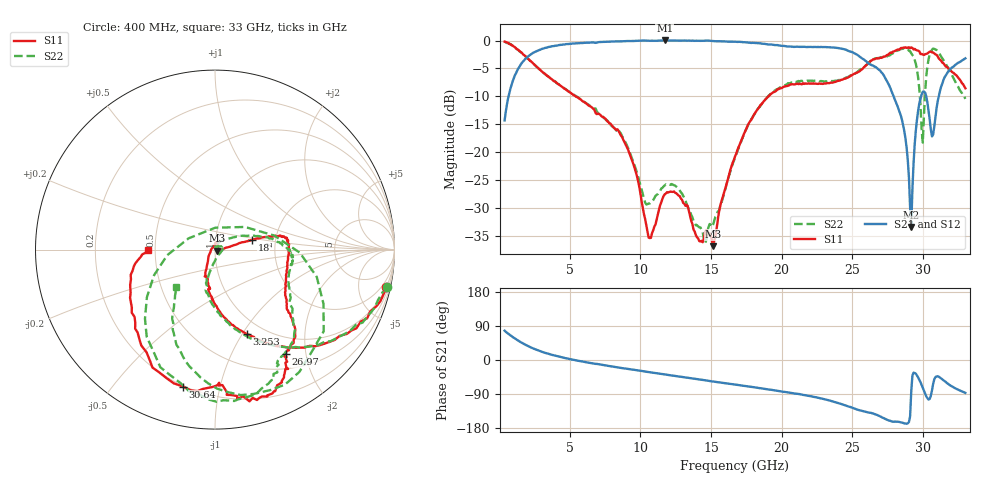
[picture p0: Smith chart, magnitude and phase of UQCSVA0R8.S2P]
!  Part Number  UQCSVA0R8  Mounting Orientation: Horizontal
!  Description: Ultra Low ESR Microwave capacitors
!  Application: Coupling, Bypass, Tuning, DC Block
!  Filters, Matching
# GHZ S DB R 50
! Freq  |S11|  S11 Ph  |S21|  S21 Ph  |S12|  S12 Ph  |S22|  S22 Ph
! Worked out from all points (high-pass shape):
!   401 points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, 400 MHz to 33 GHz, reference 50 ohm
!   highest |S21| = 0.01 dB at 11.73 GHz (marker M1); lowest = -33.4 dB at 29.17 GHz (marker M2)
!   |S21| within 3 dB of the highest: 2.002 GHz to 25.57 GHz (23.57 GHz wide, 171 % of centre)
!   lowest |S11| = -36.8 dB at 15.15 GHz (marker M3), VSWR 1.03, Z = 51.3 - j0.652 ohm
!   |S11| at or under -10 dB: 5.422 GHz to 19.08 GHz (13.66 GHz wide, 111 % of centre)
!   |S22| runs from -36.4 to -0.2 dB; largest |S21 - S12| = 0.01
!   S11 on the Smith chart (normalised r, x): 400 MHz: 0.92, -9.07; 3.253 GHz: 0.83, -1.05; 18 GHz: 1.51, +0.17; 26.97 GHz: 0.72, -1.65; 30.64 GHz: 0.20, -0.78; 33 GHz: 0.46, -0.00
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0.4  -0.19 -12.5  -14.30 77.4  -14.31 77.3  -0.17 -12.2
1.46  -1.90 -40.8  -4.66 48.9  -4.65 49.1  -1.96 -40.0
3.253  -5.98 -69.5  -1.33 19.1  -1.34 19.0  -5.98 -71.1
5.861  -10.74 -91.5  -0.46 -3.8  -0.45 -3.8  -10.66 -94.5
8.876  -18.18 -113.9  -0.12 -22.2  -0.14 -22.3  -17.89 -103.2
10.588  -35.28 150.7  -0.05 -31.9  -0.06 -31.9  -29.16 -36.3
11.321  -30.30 91.5  -0.02 -35.6  -0.04 -35.7  -27.20 3.9
11.729  -27.54 80.7  0.01 -38.0  -0.01 -38.0  -25.93 13.6
15.152  -36.82 -26.1  -0.11 -56.8  -0.11 -56.8  -32.96 81.5
16.7  -20.76 12.1  -0.21 -64.7  -0.22 -64.6  -20.94 40.7
18.004  -13.45 14.8  -0.42 -71.6  -0.43 -71.7  -13.45 21.7
22.161  -7.75 -1.7  -1.17 -96.2  -1.15 -96.1  -7.20 -8.3
26.969  -3.06 -55.9  -5.40 -149.0  -5.42 -148.6  -3.08 -58.3
27.621  -2.31 -58.8  -8.11 -160.1  -8.13 -160.1  -2.67 -61.8
28.599  -1.28 -68.3  -15.20 -166.1  -15.19 -166.8  -1.47 -81.2
29.17  -1.24 -77.2  -33.38 -82.8  -32.77 -86.2  -2.29 -104.5
29.659  -1.81 -85.4  -12.51 -46.2  -12.55 -46.5  -6.68 -145.0
29.985  -2.49 -88.1  -9.18 -73.3  -9.23 -73.5  -18.28 89.5
30.311  -2.32 -91.1  -11.06 -100.6  -11.04 -100.4  -4.63 -15.0
30.637  -2.12 -103.1  -17.17 -80.1  -17.00 -80.5  -1.64 -55.4
31.452  -4.07 -135.3  -7.01 -53.7  -6.99 -53.0  -3.53 -102.3
33  -8.56 -179.3  -3.19 -86.8  -3.16 -86.9  -10.44 -136.8
